{attribute 'TcDependDnClassFactory ' := 'DataConvertDrv'}
FUNCTION_BLOCK FB_DynProxyTcComConvertModule EXTENDS FB_DynProxyTcComModule
VAR_INPUT
END_VAR
VAR_OUTPUT
END_VAR
VAR
	_iThisProvider		: IAnalogToPWM;
END_VAR

METHOD FB_exit : BOOL
VAR_INPUT
	bInCopyCode : BOOL; // if TRUE, the exit method is called for exiting an instance that is copied afterwards (online change).
END_VAR
IF NOT bInCopyCode THEN
	FW_SafeRelease(pipUnk:= ADR(_iThisProvider));
END_IF
END_METHOD

METHOD FB_init : BOOL
VAR_INPUT
	bInitRetains 	: BOOL; // if TRUE, the retain variables are initialized (warm start / cold start)
	bInCopyCode 	: BOOL;  // if TRUE, the instance afterwards gets moved into the copy code (online change)
	classID			: CLSID;
	IID				: IID;
	sObjectName		: STRING;
	eObjState		: TCOM_STATE;
END_VAR
ComQueryInterface(Super^._iProvider,TC_GLOBAL_IID_LIST.IID_IAnalogToPWM, ADR(_iThisProvider));
END_METHOD

PROPERTY ip : IAnalogToPWM
GET
ip	:= _iThisProvider;
END_GET
END_PROPERTY

END_FUNCTION_BLOCK
